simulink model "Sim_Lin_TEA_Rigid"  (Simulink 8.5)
settings: Solver=ode23  StartTime=0.0  StopTime=108000  MaxStep=1  RelTol=1e-3
InitFcn:
  | start
StopFcn:
  | pl2
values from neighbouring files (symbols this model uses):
  Kpqr = lqr(sys,Q0,R0)    [des.m]
  wo = 0.0011    [start.m]    (also in start1.m; start2.m; start3.m)
undefined symbols (not defined in the file or in its folder): Av, Bv, Cv, Dv

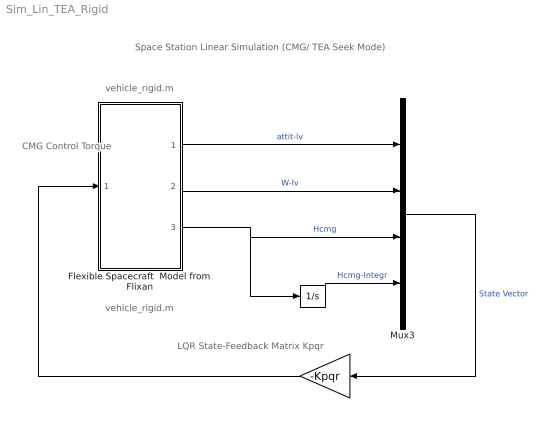
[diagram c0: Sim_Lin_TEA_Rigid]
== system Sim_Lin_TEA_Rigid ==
  note: Space Station Linear Simulation (CMG/ TEA Seek Mode)
  note: LQR State-Feedback Matrix Kpqr
  note: CMG Control Torque
  note: vehicle_rigid.m
  note: vehicle_rigid.m
  " " : Gain  Gain=-Kpqr  Multiplication=Matrix(K*u)
  "  " : Integrator
  Flexible Spacecraft  Model from Flixan : Subsystem
  Mux3 : Mux  Inputs=[3, 3, 3, 3]
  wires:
  "  "/1 -> Mux3/4  "Hcmg-Integr"
  Mux3/1 -> " "/1  "State Vector"
  Flexible Spacecraft  Model from Flixan/3("Hcmg ") -> Mux3/3, "  "/1  "Hcmg"
  " "/1 -> Flexible Spacecraft  Model from Flixan/1(Tcmg)
  Flexible Spacecraft  Model from Flixan/1(att-lv) -> Mux3/1  "attit-lv"
  Flexible Spacecraft  Model from Flixan/2(w-lv) -> Mux3/2  "W-lv"

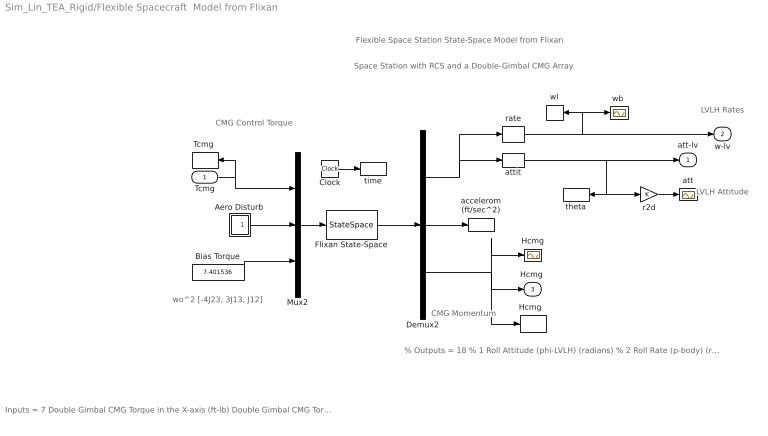
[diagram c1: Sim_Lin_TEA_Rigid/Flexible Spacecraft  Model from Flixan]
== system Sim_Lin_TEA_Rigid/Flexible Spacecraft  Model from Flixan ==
  note: Flexible Space Station State-Space Model from Flixan
  note: Space Station with RCS and a Double-Gimbal CMG Array
  note: wo^2 [-4J23, 3J13, J12]
  note: Inputs = 7 Double Gimbal CMG Torque in the X-axis (ft-lb) Double Gimbal CMG Torque in the Y-axis (ft-lb) Double Gimbal CMG Torque in the Z-axis (ft-lb) External Torque Input 1 (ft-lb), direct: External Torque Input 2 (ft-lb), direct: External Torque Input 3 (ft-lb), direct: Ext Torque Direct.=(0.197, -0.5964, -0.7782)
  note: CMG Momentum
  note: LVLH Attitude
  note: LVLH Rates
  note: CMG Control Torque
  note: % Outputs = 18 % 1 Roll Attitude (phi-LVLH) (radians) % 2 Roll Rate (p-body) (rad/sec) % 3 Pitch Attitude (thet-LVLH) (radians) % 4 Pitch Rate (q-body) (rad/sec) % 5 Yaw Attitude (psi-LVLH) (radians) % 6 Yaw Rate (r-body) (rad/sec) % 7 Angle of attack, alfa, (radians) % 8 Angle of sideslip, beta, (radian) % 9 Change in Altitude, delta-h, (feet) % 10 Forward Acceleration (V-dot) (ft/sec) % 11 Cross Range Velocity (Vcr) (ft/sec) % 12 Accelerom # 1, (along X), (ft/sec^2) Translat. Acceler % 13 Accelerom # 2, (along Z), (ft/sec^2) Translat. Acceler % 14 Accelerom # 3, (along X), (ft/sec^2) Translat. Acceler % 15 Accelerom # 4, (along Z), (ft/sec^2) Translat. Acceler % 16 Double Gimbal CMG Momentum Change in X-axis (ft-lb-sec) % 17 Double Gimbal CMG Momentum Change in Y-axis (ft-lb-sec) % 18 Double Gimbal CMG Momentum Change in Z-axis (ft-lb-sec)
  Tcmg : Inport  PortDimensions=3
  Aero Disturb : Subsystem
  Bias Torque : Constant  Value=7.401536
  Clock : Clock
  Demux2 : Demux  Outputs=[11, 4, 3]
  Flixan State-Space : StateSpace  A=Av  B=Bv  C=Cv  D=Dv  X0=0
  Hcmg : Scope
  "Hcmg  " : ToWorkspace  VariableName=Hcmg  SampleTime=-1
  Mux2 : Mux  Inputs=[3, 3, 1]
  "Tcmg " : ToWorkspace  VariableName=Tcmg  SampleTime=-1
  accelerom (ft/sec^2) : ToWorkspace  VariableName=accel  SampleTime=-1
  att : Scope
  attit : Selector  InputPortWidth=11  Indices=[1,3,5]
  r2d : Gain
  rate : Selector  InputPortWidth=11  Indices=[2, 4, 6]
  theta : ToWorkspace  VariableName=theta  SampleTime=-1
  time : ToWorkspace  VariableName=time  SampleTime=-1
  "wb " : Scope
  wl : ToWorkspace  VariableName=wl  SampleTime=-1
  att-lv : Outport
  w-lv : Outport  Port=2
  "Hcmg " : Outport  Port=3
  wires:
  Mux2/1 -> Flixan State-Space/1
  Clock/1 -> time/1
  Demux2/3 -> "Hcmg  "/1, Hcmg/1, "Hcmg "/1
  Demux2/2 -> accelerom (ft/sec^2)/1
  attit/1 -> att-lv/1, r2d/1, theta/1
  Tcmg/1 -> Mux2/1, "Tcmg "/1
  Flixan State-Space/1 -> Demux2/1
  Demux2/1 -> attit/1, rate/1
  rate/1 -> w-lv/1, wl/1, "wb "/1
  r2d/1 -> att/1
  Aero Disturb/1(Td) -> Mux2/2
  Bias Torque/1 -> Mux2/3

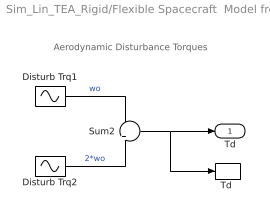
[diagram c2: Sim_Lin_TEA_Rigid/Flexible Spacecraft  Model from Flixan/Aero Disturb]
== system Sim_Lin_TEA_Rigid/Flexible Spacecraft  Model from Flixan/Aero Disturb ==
  note: Aerodynamic Disturbance Torques
  Disturb Trq1 : Sin  Amplitude=[1, 3, 1]  Bias="[1  8  1]"  Frequency=[wo, wo, wo]  SampleTime=0
  Disturb Trq2 : Sin  Amplitude=[1, 1, 1]*0.5  Frequency=[wo, wo, wo]*2  SampleTime=0
  Sum2 : Sum  Inputs=+|+
  "Td " : ToWorkspace  VariableName=Td  SampleTime=-1
  Td : Outport
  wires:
  Disturb Trq1/1 -> Sum2/1  "wo"
  Sum2/1 -> Td/1, "Td "/1
  Disturb Trq2/1 -> Sum2/2  "2*wo"
